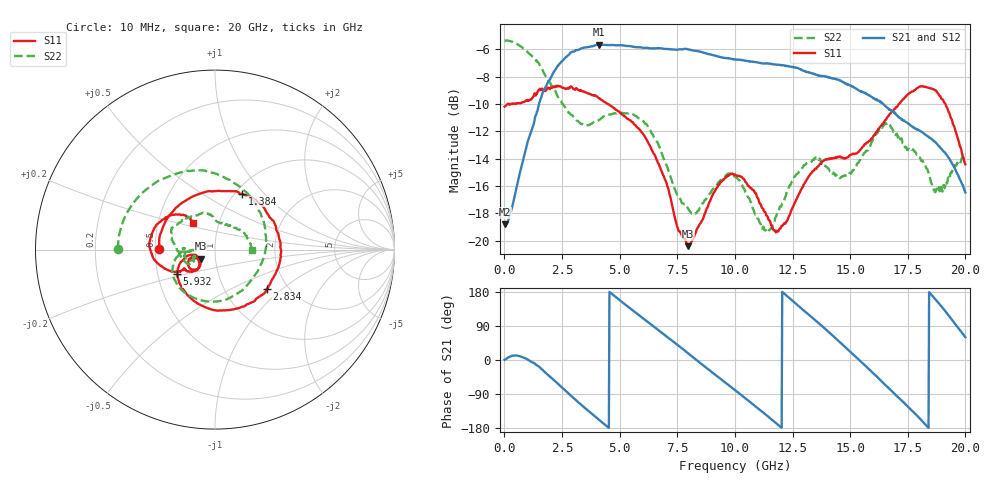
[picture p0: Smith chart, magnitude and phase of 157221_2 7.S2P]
!  2-Port S-parameters saved by WinCal
! VAR MeasName=S-Parameters (CALIBRATED_DATA) read from VNA (N5242A)
! VAR MeasDate=2015-5-26 16:47:40
! VAR NAME=157221_2 7
! VAR FILENAME=157221_2 7.S2P
! VAR DATE=2015-5-26 16:47:40
! VAR PHYS_PORTS=1,2
# Hz S DB R 50
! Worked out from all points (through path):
!   801 points, 10 MHz to 20 GHz, reference 50 ohm
!   highest |S21| = -5.64 dB at 4.108 GHz (marker M1); lowest = -18.8 dB at 10 MHz (marker M2)
!   lowest |S11| = -20.4 dB at 7.981 GHz (marker M3), VSWR 1.21, Z = 42.3 - j4.34 ohm
!   |S11| at or under -10 dB: start of sweep to 141.3 MHz; 4.499 GHz to 17.12 GHz (12.62 GHz wide, 117 % of centre); 19.13 GHz to end of sweep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
!   |S22| runs from -19.3 to -5.3 dB; largest |S21 - S12| = 0.0083
!   S11 on the Smith chart (normalised r, x): 10 MHz: 0.53, +0.00; 1.384 GHz: 1.07, +0.76; 2.834 GHz: 1.57, -0.79; 5.932 GHz: 0.63, -0.18; 20 GHz: 0.75, +0.23
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1e7  -10.19 179.4  -18.81 0.4  -18.80 0.5  -5.36 179.6
7.346375e8  -9.90 116.8  -14.63 8.7  -14.61 8.6  -5.80 141.4
1.384312e9  -9.22 64.3  -10.77 -12.4  -10.76 -12.5  -6.78 105.5
2.083962e9  -8.80 9.1  -7.82 -49.2  -7.81 -49.4  -8.72 62.8
2.833588e9  -8.82 -37.0  -6.31 -90.5  -6.30 -90.7  -10.67 13.6
3.358325e9  -9.05 -64.3  -5.91 -119.4  -5.89 -119.7  -11.46 -22.3
4.10795e9  -9.59 -94.4  -5.64 -157.9  -5.64 -158.1  -11.17 -67.2
4.957525e9  -10.54 -120.4  -5.69 160.3  -5.69 160.1  -10.68 -107.9
5.932038e9  -12.02 -147.1  -5.85 113.8  -5.87 113.6  -11.10 -146.1
6.681662e9  -14.36 -161.1  -5.90 78.9  -5.88 78.8  -12.97 -166.9
7.981012e9  -20.41 -147.8  -5.99 17.2  -5.98 16.9  -17.69 -168.9
8.855575e9  -17.36 -131.8  -6.34 -25.1  -6.31 -25.5  -16.71 -155.2
1.0005e10  -15.16 -147.4  -6.73 -79.4  -6.73 -79.9  -15.32 -170.4
1.087956e10  -16.52 -160.4  -6.92 -121.7  -6.90 -121.9  -18.10 -179.2
1.18041e10  -19.36 -150.0  -7.12 -167.5  -7.09 -168.2  -18.17 -157.7
1.335332e10  -14.97 -136.2  -7.76 111.7  -7.70 111.6  -14.16 -170.2
1.42029e10  -14.00 -145.8  -8.08 66.7  -8.08 65.9  -15.00 178.7
1.512744e10  -13.63 -147.6  -8.72 14.7  -8.70 14.5  -14.86 -175.5
1.667666e10  -10.85 -156.8  -10.36 -74.8  -10.34 -75.0  -11.48 152.4
1.827586e10  -8.74 170.6  -12.25 -171.0  -12.24 -172.0  -14.58 94.6
1.92004e10  -10.25 140.9  -13.76 123.4  -13.78 122.4  -15.82 49.7
2e10  -14.42 129.7  -16.48 60.2  -16.53 59.0  -13.66 -0.5
